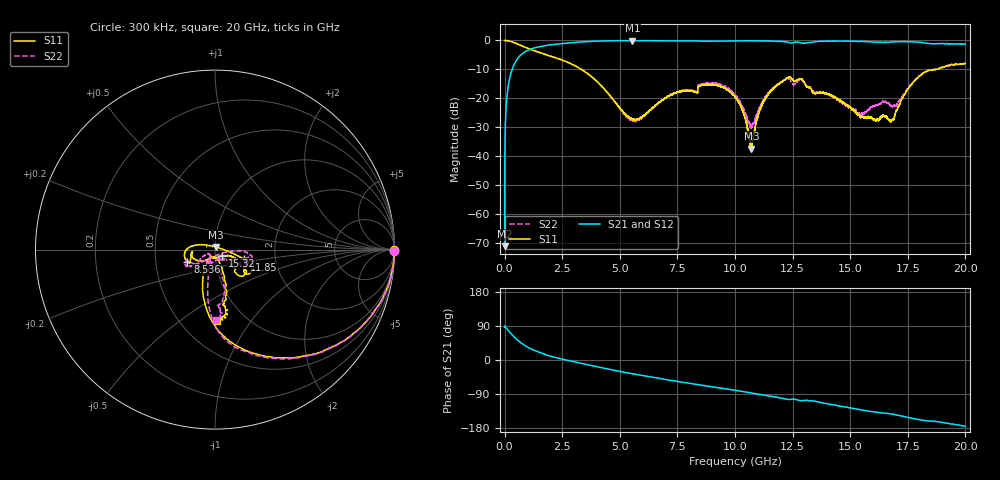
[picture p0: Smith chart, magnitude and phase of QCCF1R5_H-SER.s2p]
!{QCCF1R5}
!Johanson Technology Inc.
!www.johansontechnology.com
!Test Board Conditions:
!Substrate Type  RO4350B
!Substrate Thickness  10 mil
!Substrate Dk  3.66
!TL Type: GCPW
!TL Trace Width  21 mil
!TL Gap  20 mil
!Electrode orientation  Horizontal
!DUT TOPOLOGY	SERIES
!Mounting Pad LxW  16x21 mil
! Created Sat Jan  9 18:10:24 2021
# hz S ma R 50
! 2 Port Network Data from SP1.SP block
! freq  magS11  angS11  magS21  angS21  magS12  angS12  magS22  angS22
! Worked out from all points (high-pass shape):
!   20001 points, 300 kHz to 20 GHz, reference 50 ohm
!   highest |S21| = -0.07 dB at 5.547 GHz (marker M1); lowest = -71.0 dB at 300 kHz (marker M2)
!   |S21| within 3 dB of the highest: 1.111 GHz to end of sweep
!   lowest |S11| = -37.3 dB at 10.71 GHz (marker M3), VSWR 1.03, Z = 50.5 + j1.28 ohm
!   |S11| at or under -10 dB: 3.333 GHz to 18.72 GHz (15.39 GHz wide, 140 % of centre); 18.72537 GHz to 18.73069 GHz (5.323 MHz wide, 0.0284 % of centre); 18.73303 GHz to 18.73338 GHz (348.1 kHz wide, 0.00186 % of centre)
!   |S22| runs from -30.3 to 0.0 dB; largest |S21 - S12| = 0.013
!   S11 on the Smith chart (normalised r, x): 300 kHz: open; 8.536 GHz: 0.73, -0.10; 11.85 GHz: 1.38, -0.16; 15.32 GHz: 1.08, -0.07; 20 GHz: 0.75, -0.70
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300000  0.9987 -0.3  0.000282 86.4  0.0003111 96.8  0.9989 -0.4
1.013e8  0.9917 -7.4  0.1048 82.3  0.105 82.3  0.9913 -7.5
1.273e8  0.9906 -9.3  0.1315 80.3  0.1315 80.4  0.9903 -9.3
2.523e8  0.9648 -18.1  0.2525 71.3  0.252 71.2  0.9655 -18.2
4.633e8  0.9008 -31.4  0.4217 58.1  0.4217 58.0  0.9012 -31.6
1.8503e9  0.5574 -76.4  0.8238 12.5  0.8235 12.6  0.5592 -78.0
3.3343e9  0.3162 -99.7  0.9428 -8.9  0.9421 -8.9  0.3172 -96.3
5.5473e9  0.04331 -120.8  0.9919 -36.3  0.9904 -36.3  0.04063 -132.6
6.6673e9  0.083 -133.1  0.9875 -48.2  0.9876 -48.2  0.08406 -149.5
8.5363e9  0.1683 -156.2  0.9743 -66.4  0.9755 -66.4  0.176 -157.0
1.00003e10  0.1063 165.9  0.9825 -80.0  0.9811 -80.0  0.1153 -139.0
1.03573e10  0.05841 153.7  0.9863 -83.4  0.985 -83.5  0.06886 -127.5
1.07083e10  0.01365 68.2  0.986 -87.1  0.9853 -87.0  0.03143 -70.6
1.11573e10  0.07533 -7.1  0.9831 -91.6  0.982 -91.6  0.0814 -8.2
1.18453e10  0.1721 -18.5  0.968 -98.7  0.9679 -98.8  0.1765 -5.0
1.28443e10  0.2155 -38.8  0.913 -107.3  0.9133 -107.3  0.2105 -21.6
1.33343e10  0.1357 -44.0  0.9243 -107.6  0.9255 -107.7  0.1413 -31.1
1.53183e10  0.05207 -39.9  0.9627 -129.8  0.9633 -129.8  0.05508 -68.3
1.66673e10  0.04334 -111.0  0.9269 -141.1  0.9282 -141.3  0.08379 -122.6
1.69543e10  0.05416 -79.0  0.9506 -144.4  0.9526 -144.3  0.07552 -98.2
1.81753e10  0.2745 -77.6  0.9136 -159.5  0.9153 -159.2  0.2714 -79.5
2e10  0.3966 -88.1  0.8661 -175.2  0.8621 -175.0  0.3933 -89.5
